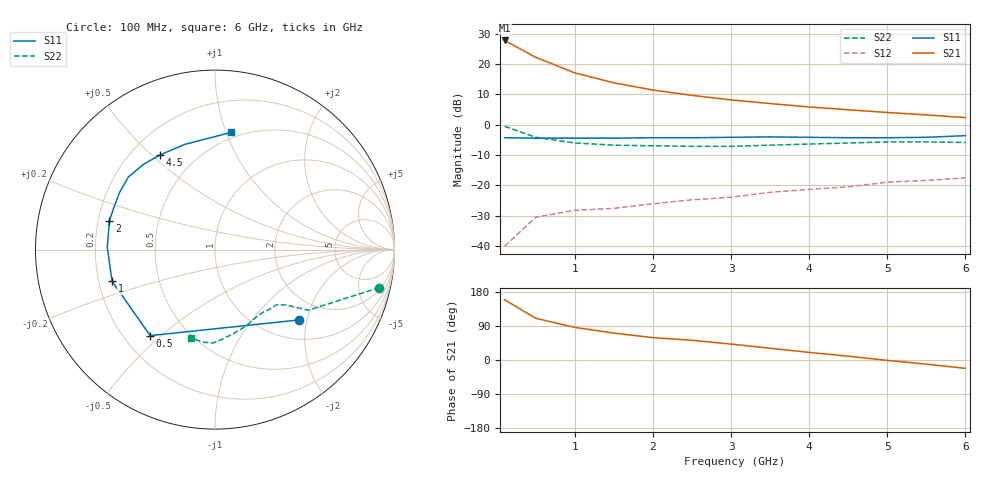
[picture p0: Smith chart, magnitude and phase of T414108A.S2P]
!AT-41410
!S-PARAMETERS at Vce=8V  Ic=10mA.  LAST UPDATED 07-21-92
# ghz s ma r 50
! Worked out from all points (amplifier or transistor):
!   13 points, 100 MHz to 6 GHz, reference 50 ohm
!   highest |S21| = 27.7 dB at 100 MHz (marker M1)
!   |S21| within 3 dB of that: start of sweep to 315.2 MHz
!   unconditionally stable (mu >= 1): 1.393 GHz to 5.98 GHz
!   at 1 GHz: K = 0.77, MSG = 22.6 dB, |S12| = -28.2 dB
!   at 3 GHz: K = 1.32, MAG = 12.6 dB, |S12| = -23.9 dB
!   at 6 GHz: K = 1.00, MSG = 9.9 dB, |S12| = -17.5 dB
!   lowest NFmin = 1.20 dB at 100 MHz
!   S11 on the Smith chart (normalised r, x): 100 MHz: 1.44, -1.79; 500 MHz: 0.31, -0.46; 1 GHz: 0.26, -0.14; 2 GHz: 0.25, +0.12; 4.5 GHz: 0.32, +0.53; 6 GHz: 0.45, +1.04
0.1  0.61 -40.0  24.38 159.0  0.01 75.0  0.94 -13.0
0.5  0.6 -127.0  12.83 110.0  0.03 40.0  0.62 -33.0
1  0.6 -163.0  7.12 86.0  0.039 35.0  0.5 -38.0
1.5  0.6 179.0  4.89 71.0  0.042 45.0  0.46 -42.0
2  0.61 165.0  3.72 59.0  0.05 42.0  0.45 -48.0
2.5  0.61 158.0  3.04 52.0  0.058 46.0  0.44 -52.0
3  0.62 149.0  2.56 42.0  0.064 50.0  0.44 -58.0
3.5  0.63 140.0  2.23 31.0  0.077 48.0  0.46 -68.0
4  0.62 130.0  1.96 20.0  0.086 44.0  0.48 -78.0
4.5  0.61 120.0  1.76 10.0  0.095 41.0  0.5 -85.0
5  0.61 106.0  1.59 -1.0  0.113 38.0  0.52 -91.0
5.5  0.62 94.0  1.45 -11.0  0.121 33.0  0.52 -97.0
6  0.66 82.0  1.31 -22.0  0.133 30.0  0.51 -105.0
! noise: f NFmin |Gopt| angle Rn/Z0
0.1  1.2  0.12  4  0.17
0.5  1.2  0.1  23  0.17
1  1.3  0.06  49  0.16
2  1.6  0.26  172  0.16
4  3  0.46  -133  0.26
